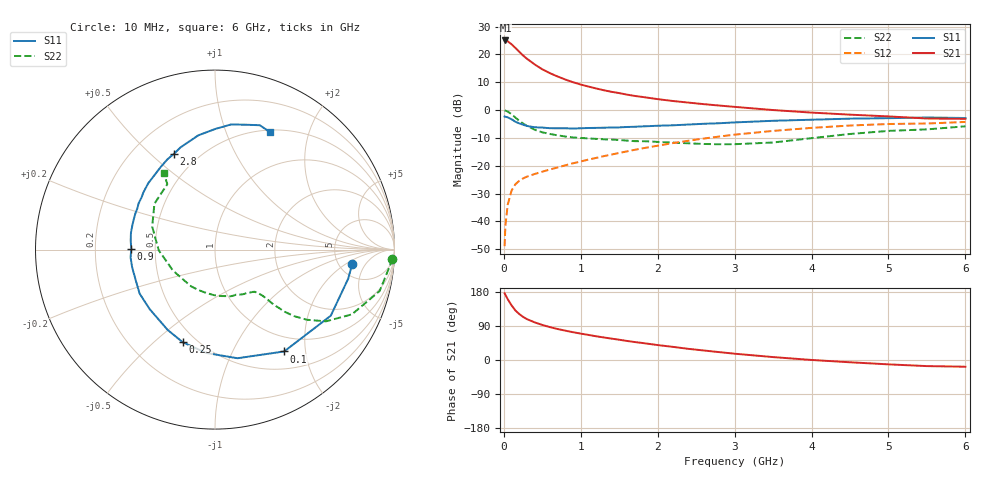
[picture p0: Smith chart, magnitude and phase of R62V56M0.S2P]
! SIEMENS Small Signal Semiconductors
! BFR193
! Si NPN RF Bipolar Junction Transistor in SOT23
! VCE = 2.5 V  IC = 6 mA
! Common Emitter S-Parameters:  May  1996
# GHz  S  MA  R  50
!  f  S11  S21  S12  S22
! GHz  MAG  ANG  MAG  ANG  MAG  ANG  MAG  ANG
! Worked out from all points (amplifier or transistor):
!   36 points, 10 MHz to 6 GHz, reference 50 ohm
!   highest |S21| = 25.0 dB at 20 MHz (marker M1)
!   |S21| within 3 dB of that: start of sweep to 161.4 MHz
!   unconditionally stable (mu >= 1): 850.6 MHz to 1.979 GHz
!   at 250 MHz: K = 0.48, MSG = 22.1 dB, |S12| = -24.5 dB
!   at 1.4 GHz: K = 1.06, MAG = 9.8 dB, |S12| = -16.0 dB
!   at 6 GHz: K = 0.96, MSG = 0.6 dB, |S12| = -4.3 dB
!   lowest NFmin = 1.20 dB at 450 MHz
!   S11 on the Smith chart (normalised r, x): 10 MHz: 6.57, -2.62; 100 MHz: 0.76, -1.62; 250 MHz: 0.42, -0.62; 900 MHz: 0.36, +0.00; 2.8 GHz: 0.37, +0.60; 6 GHz: 0.53, +1.44
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0.01  0.7684 -6.1  17.73 176.3  0.0036 86.7  0.9899 -2.9
0.02  0.7597 -12.3  17.84 171.9  0.0082 84.8  0.9767 -5.7
0.05  0.7428 -29.7  17.26 160.7  0.0199 75.4  0.946 -14.1
0.1  0.686 -55.8  15.23 144.3  0.0358 64.6  0.844 -25.3
0.15  0.6181 -78.3  13.09 130.7  0.0465 57.2  0.7359 -32.9
0.2  0.578 -94.8  11.17 121.4  0.0537 53.0  0.6435 -37.4
0.25  0.5467 -109.1  9.576 113.8  0.0593 50.4  0.575 -40.1
0.3  0.5196 -120.5  8.379 107.9  0.0638 49.5  0.5212 -41.7
0.4  0.4923 -137.7  6.629 99.4  0.0711 49.4  0.4447 -43.2
0.5  0.4863 -149.8  5.404 92.5  0.0784 50.3  0.3993 -43.6
0.6  0.4732 -159.3  4.603 86.7  0.086 51.7  0.3727 -44.0
0.7  0.472 -168.0  4.012 81.7  0.0933 53.4  0.3518 -44.8
0.9  0.4667 179.4  3.169 73.3  0.111 56.2  0.323 -46.7
1.1  0.4775 168.8  2.649 66.2  0.1293 58.0  0.3102 -50.3
1.3  0.4829 159.7  2.275 59.5  0.1492 58.8  0.2987 -54.2
1.6  0.4979 148.6  1.899 50.3  0.1816 59.1  0.2836 -62.2
2.2  0.5338 129.5  1.456 34.6  0.2561 55.7  0.2608 -82.8
2.8  0.5812 113.1  1.208 20.8  0.3353 49.1  0.2437 -112.1
3.5  0.6435 98.3  1.003 7.7  0.4234 38.3  0.262 -153.6
4.5  0.7029 82.7  0.829 -6.0  0.5287 22.1  0.3727 159.9
5.5  0.7365 70.2  0.707 -16.1  0.5752 5.5  0.4509 126.1
6  0.722 64.7  0.697 -17.7  0.6129 0.7  0.5117 123.8
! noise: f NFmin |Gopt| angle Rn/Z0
0.45  1.2  0.25  114  0.13
0.9  1.25  0.37  150  0.12
1.8  2  0.55  -158  0.12
